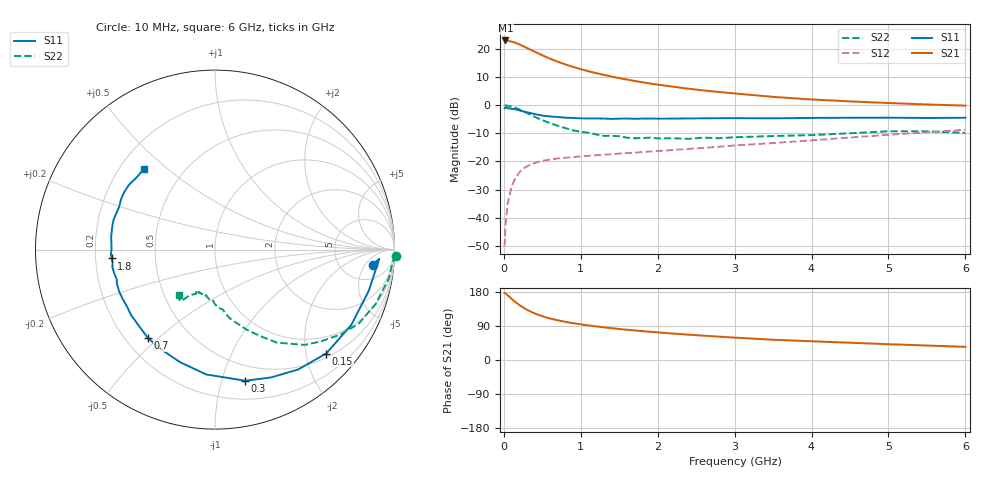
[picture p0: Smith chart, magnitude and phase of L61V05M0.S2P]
!  INFINEON TECHNOLOGIES Small Signal Semiconductors
! BFR380L3 , Si-NPN RF-Transistor in TSLP-3-1
!  Vce=1 V,  Ic=5 mA
! Common Emitter S-Parameters:  07. March 2005
#  GHz  S  MA  R  50
! f  S11  S21  S12  S22
! GHz  Mag  Ang  Mag  Ang  Mag  Ang  Mag  Ang
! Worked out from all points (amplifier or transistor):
!   36 points, 10 MHz to 6 GHz, reference 50 ohm
!   highest |S21| = 23.1 dB at 20 MHz (marker M1)
!   |S21| within 3 dB of that: start of sweep to 324.1 MHz
!   unconditionally stable (mu >= 1): 2.324 GHz to 4.882 GHz
!   at 250 MHz: K = 0.18, MSG = 21.9 dB, |S12| = -22.7 dB
!   at 1.4 GHz: K = 0.78, MSG = 13.8 dB, |S12| = -17.4 dB
!   at 6 GHz: K = 0.97, MSG = 4.3 dB, |S12| = -8.7 dB
!   S11 on the Smith chart (normalised r, x): 10 MHz: 10, -8; 150 MHz: 0.59, -2.41; 300 MHz: 0.36, -1.19; 700 MHz: 0.29, -0.46; 1.8 GHz: 0.27, -0.04; 6 GHz: 0.30, +0.41
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0.01  0.8828 -5.4  14.22 176.5  0.0031 86.3  1.01 -1.9
0.02  0.9165 -3.2  14.23 176.6  0.0069 85.6  0.9922 -3.9
0.05  0.8871 -15.0  14.06 170.5  0.0177 82.8  0.9811 -9.5
0.1  0.8675 -29.0  13.58 161.6  0.0356 75.9  0.9455 -18.6
0.15  0.8478 -43.1  12.96 152.9  0.0507 67.8  0.9006 -27.3
0.2  0.8127 -55.3  12.14 145.2  0.0636 62.8  0.8437 -34.1
0.25  0.7778 -66.3  11.29 138.7  0.0733 57.2  0.78 -41.0
0.3  0.7498 -77.0  10.45 132.5  0.0818 53.4  0.7286 -46.8
0.4  0.6974 -94.0  8.986 122.9  0.0937 47.3  0.6221 -56.4
0.5  0.6566 -107.3  7.75 115.6  0.1025 43.4  0.5414 -62.6
0.6  0.6313 -118.8  6.735 109.5  0.108 40.9  0.4807 -68.3
0.7  0.6184 -127.2  5.965 104.8  0.1128 39.6  0.4312 -73.1
0.9  0.593 -142.1  4.809 97.1  0.1191 38.0  0.356 -81.1
1.1  0.5831 -151.8  4.031 91.2  0.1261 38.5  0.3239 -86.8
1.4  0.5721 -163.2  3.233 84.1  0.1342 39.8  0.2858 -93.3
1.8  0.5782 -175.1  2.571 76.1  0.1466 42.7  0.2605 -101.4
2.2  0.5782 176.6  2.137 69.7  0.16 46.0  0.2584 -106.3
2.8  0.5878 165.9  1.72 61.6  0.1825 50.2  0.2586 -114.1
3.5  0.5848 156.0  1.409 53.4  0.2125 53.0  0.283 -117.5
4.5  0.5987 147.7  1.171 45.6  0.2664 56.7  0.317 -121.3
5.5  0.5937 137.6  1.033 38.2  0.3307 56.6  0.3427 -125.5
6  0.5988 131.7  0.985 34.7  0.3661 55.6  0.3229 -128.9
